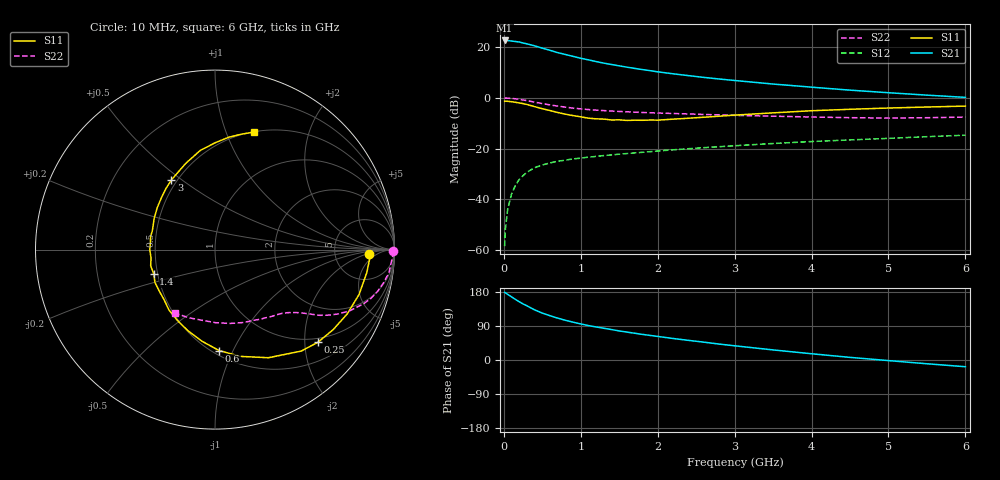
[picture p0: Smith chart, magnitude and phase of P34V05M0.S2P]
! SIEMENS Small Signal Semiconductors
! BFP181
! Si NPN RF Bipolar Junction Transistor in SOT143
! VCE = 4 V  IC = 5 mA
! Common Emitter S-Parameters:  March  1996
# GHz  S  MA  R  50
!  f  S11  S21  S12  S22
! GHz  MAG  ANG  MAG  ANG  MAG  ANG  MAG  ANG
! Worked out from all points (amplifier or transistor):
!   36 points, 10 MHz to 6 GHz, reference 50 ohm
!   highest |S21| = 22.6 dB at 10 MHz (marker M1)
!   |S21| within 3 dB of that: start of sweep to 496.1 MHz
!   unconditionally stable (mu >= 1): 1.723 GHz to end of sweep
!   at 250 MHz: K = 0.22, MSG = 26.1 dB, |S12| = -30.6 dB
!   at 1.4 GHz: K = 0.90, MSG = 17.8 dB, |S12| = -22.5 dB
!   at 6 GHz: K = 1.05, MAG = 6.0 dB, |S12| = -14.7 dB
!   lowest NFmin = 1.55 dB at 450 MHz
!   S11 on the Smith chart (normalised r, x): 10 MHz: 12, -3; 250 MHz: 0.90, -2.30; 600 MHz: 0.54, -0.89; 1.4 GHz: 0.48, -0.15; 3 GHz: 0.47, +0.46; 6 GHz: 0.50, +1.26
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0.01  0.857 -1.8  13.52 178.5  0.0012 86.1  0.991 -0.6
0.02  0.8624 -3.8  13.49 177.5  0.0026 87.2  0.9925 -1.5
0.05  0.8554 -8.6  13.49 173.2  0.0064 87.3  0.9855 -3.8
0.1  0.8407 -17.3  13.17 166.6  0.0127 79.1  0.9775 -7.6
0.2  0.7952 -34.1  12.61 153.7  0.0247 71.8  0.9355 -14.4
0.25  0.7716 -42.0  12.03 147.9  0.0294 67.6  0.9089 -17.5
0.3  0.7416 -49.7  11.6 143.0  0.0343 64.3  0.8828 -19.9
0.4  0.672 -63.7  10.6 132.3  0.0422 58.5  0.8247 -24.4
0.5  0.6116 -76.6  9.532 123.7  0.0475 53.4  0.7723 -27.7
0.6  0.5633 -87.6  8.65 116.8  0.0524 50.1  0.7267 -30.2
0.7  0.5154 -98.2  7.782 110.5  0.0565 47.8  0.6889 -32.1
0.8  0.4771 -108.3  7.153 104.8  0.0593 45.3  0.6571 -33.4
0.9  0.4481 -117.5  6.572 99.8  0.0628 43.8  0.6292 -34.6
1.1  0.398 -135.5  5.608 90.8  0.0681 41.5  0.5888 -36.7
1.4  0.3671 -158.5  4.539 80.3  0.0754 39.9  0.5506 -39.6
1.8  0.3618 174.1  3.615 67.6  0.0848 38.6  0.5155 -43.6
2.2  0.3808 152.9  2.98 56.8  0.0947 37.2  0.4927 -48.5
3  0.4575 122.2  2.201 37.5  0.1141 33.6  0.4524 -60.1
3.5  0.5071 108.8  1.873 26.6  0.1263 31.1  0.4358 -68.8
4.5  0.5959 89.8  1.42 6.9  0.1486 24.8  0.4075 -89.3
5.5  0.6605 77.0  1.132 -9.9  0.1721 19.1  0.407 -111.3
6  0.6891 71.7  1.023 -17.8  0.1841 15.5  0.4184 -122.6
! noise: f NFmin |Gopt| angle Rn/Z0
0.45  1.55  0.48  17  0.36
0.9  1.65  0.4  35  0.34
1.8  2  0.18  88  0.34
